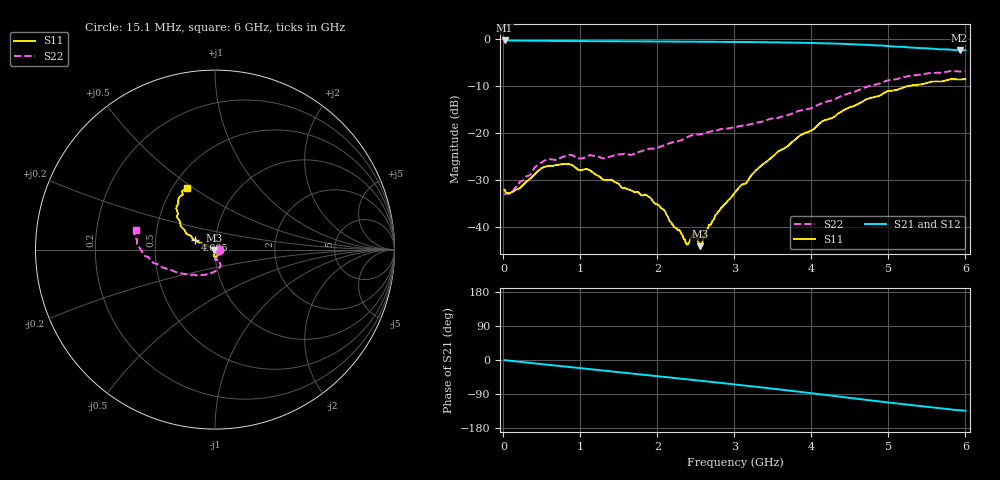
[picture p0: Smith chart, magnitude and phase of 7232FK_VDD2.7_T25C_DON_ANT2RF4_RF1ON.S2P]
!Agilent Technologies,E5071C,MY46417908,A.11.23
!Date: Fri Mar 03 11:32:10 2017
!Data & Calibration Information:
!Freq	S11:SOLT2(ON)	S21:SOLT2(ON)	S12:SOLT2(ON)	S22:SOLT2(ON)
!PortZ  Port1:50+j0  Port2:50+j0
!Above PortZ is port z conversion or system Z0 setting when saving the data.
!When reading, reference impedance value at option line is always used.
# Hz S dB R 50
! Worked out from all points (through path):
!   400 points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, 15.1 MHz to 6 GHz, reference 50 ohm
!   highest |S21| = -0.26 dB at 15.1 MHz (marker M1); lowest = -2.4 dB at 5.925 GHz (marker M2)
!   group delay of S21, straight-line fit = 62.6 ps
!   lowest |S11| = -44.2 dB at 2.55 GHz (marker M3), VSWR 1.01, Z = 49.4 - j0.183 ohm
!   |S11| at or under -10 dB: start of sweep to 5.258 GHz
!   |S22| runs from -33.3 to -6.8 dB; largest |S21 - S12| = 0.0078
!   S11 on the Smith chart (normalised r, x): 15.1 MHz: 1.05, -0.01; 4.095 GHz: 0.80, +0.09; 6 GHz: 0.59, +0.47
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1.509975e7  -32.10 -8.3  -0.26 -0.4  -0.25 -0.4  -33.27 -8.1
6.0099e7  -32.88 -18.8  -0.28 -1.4  -0.27 -1.4  -33.04 -20.8
2.100965e8  -31.80 -47.3  -0.30 -4.7  -0.29 -4.7  -30.50 -48.7
5.40091e8  -27.22 -81.1  -0.35 -11.8  -0.34 -11.8  -25.85 -79.8
8.550858e8  -26.68 -88.5  -0.38 -18.5  -0.38 -18.5  -24.68 -88.5
1.020083e9  -27.89 -92.1  -0.39 -21.9  -0.39 -22.0  -25.42 -86.0
1.665072e9  -32.32 -104.0  -0.45 -35.6  -0.45 -35.6  -24.68 -76.8
1.845069e9  -33.17 -109.3  -0.47 -39.5  -0.46 -39.4  -23.62 -76.4
2.010066e9  -35.39 -103.5  -0.48 -42.9  -0.48 -42.9  -23.14 -72.1
2.220063e9  -40.18 -108.9  -0.50 -47.4  -0.49 -47.4  -21.88 -69.8
2.295062e9  -41.00 -108.0  -0.50 -49.0  -0.50 -49.0  -21.64 -69.2
2.38506e9  -43.88 -128.1  -0.52 -51.0  -0.51 -51.0  -20.91 -70.0
2.475059e9  -41.42 -155.4  -0.52 -52.9  -0.52 -52.9  -20.37 -72.3
2.550058e9  -44.19 -162.5  -0.53 -54.5  -0.53 -54.5  -20.32 -72.1
2.670056e9  -39.62 178.0  -0.54 -57.2  -0.54 -57.1  -19.79 -75.6
3.01505e9  -32.59 158.2  -0.58 -64.7  -0.58 -64.7  -18.75 -85.6
3.57004e9  -23.94 152.7  -0.68 -77.4  -0.67 -77.3  -16.78 -108.5
4.005033e9  -19.45 155.4  -0.79 -87.7  -0.78 -87.6  -14.68 -130.8
4.095032e9  -18.13 154.1  -0.83 -90.0  -0.82 -90.0  -13.95 -135.6
5.010016e9  -11.02 139.4  -1.47 -112.4  -1.47 -112.3  -8.73 -171.0
5.925001e9  -8.60 115.4  -2.38 -132.5  -2.38 -132.3  -6.91 167.2
6e9  -8.48 114.4  -2.36 -133.9  -2.40 -133.7  -6.85 166.4
